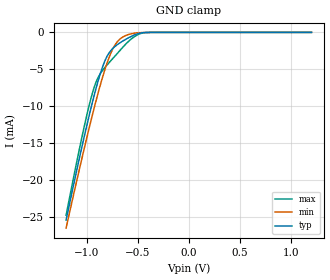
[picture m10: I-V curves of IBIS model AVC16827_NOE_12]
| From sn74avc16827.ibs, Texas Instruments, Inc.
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[Model]   AVC16827_NOE_12
Model_type  Input
Vinl=0.8
Vinh=1
| variable   typ   min   max
C_comp   2.18pF   1.38pF   2.49pF
[Temperature Range]   40   100   -40
| Ambient temperature   25   85   -40
[Voltage range]   1.2   1.2   1.2
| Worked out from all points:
|   GND clamp passes 1 mA (typ) near -0.62 V on its own axis
[GND Clamp]
| AVC16827_NOE_12
|   Voltage   I(typ)   I(min)   I(max)
-1.2V     -25.43mA   -26.52mA   -24.79mA
-1.03V    -14.59mA   -16.17mA   -13.22mA
-970mV    -11.02mA   -12.71mA   -9.647mA
-925mV    -8.519mA   -10.23mA   -7.44mA
-875mV    -6.023mA   -7.617mA   -5.813mA
-840mV    -4.552mA   -5.927mA   -5.099mA
-805mV    -3.403mA   -4.394mA   -4.511mA
-735mV    -2.07mA    -2.029mA   -3.415mA
-670mV    -1.389mA   -868.7uA   -2.401mA
-540mV    -401uA     -125uA     -658.6uA
-430mV    -25.26uA   -18.03uA   -33.69uA
1.2V      245.5pA    899.7pA    12.43pA
